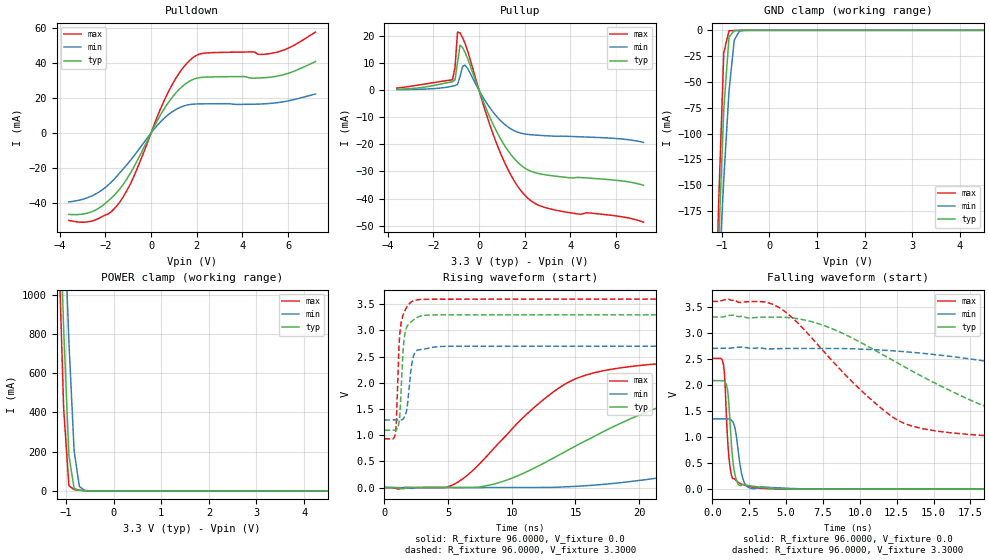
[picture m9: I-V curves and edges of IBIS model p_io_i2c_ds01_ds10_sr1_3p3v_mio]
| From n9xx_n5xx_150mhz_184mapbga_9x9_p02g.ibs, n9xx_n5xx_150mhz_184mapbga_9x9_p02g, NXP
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[Model] p_io_i2c_ds01_ds10_sr1_3p3v_mio
|   Model p_io_i2c_ds01_ds10_sr1_3p3v_mio
| This model was characterised for following simulation conditions:
| External (pad) voltage:
|   - Typ: 3.3V,   - Min: 2.7V,   - Max: 3.6V
| Library cells for typ/min/max conditions are connected as defined below:
|  pad - External Pad
|  ipp_do_lv - Core Input
|  ipp_obe_lv - Output Buffer Enable
|  IOGC - NC
|  REFH3V3 - REFH3V3
|  REFL3V3 - REFL3V3
|  ZI - NC
|  abut_ncal_vddio[1] - vddio
|  abut_ncal_vddio[2] - vddio
|  abut_ncal_vddio[3] - vssio
|  abut_ncal_vddio[4] - vddio
|  abut_ncal_vddio[5] - vddio
|  abut_ncal_vddio[6] - vssio
|  abut_pcal_vddio[1] - vssio
|  abut_pcal_vddio[2] - vssio
|  abut_pcal_vddio[3] - vddio
|  abut_pcal_vddio[4] - vssio
|  abut_pcal_vddio[5] - vssio
|  abut_pcal_vddio[6] - vddio
|  ipp_do_1p8v - ipp_do_1p8v
|  ipp_dse_lv[0] - vdd_lv
|  ipp_dse_lv[1] - 0
|  ipp_eftd_lv - NC
|  ipp_ina_mux_vddio - NC
|  ipp_ina_mux_vddio[0] - NC
|  ipp_ina_mux_vddio[1] - NC
|  ipp_ina_r0_vddio - NC
|  ipp_ina_r0a_vddio - NC
|  ipp_ina_r0b_vddio - NC
|  ipp_ina_r0c_vddio - NC
|  ipp_ina_r0d_vddio - NC
|  ipp_ina_r0e_vddio - NC
|  ipp_ina_r0f_vddio - NC
|  ipp_ina_r300_vddio - NC
|  ipp_ina_r300a_vddio - NC
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Model_type I/O
Polarity   Non-Inverting
Enable   Active-High
Vinl =   0.9900V
Vinh =   2.3100V
Vmeas =  1.6500V
Cref =   30.0000pF
Rref =   1.0000M
Vref =   3.3000V
C_comp   1.4149pF   1.3702pF   1.4746pF
|C_comp_pullup   0.5856pF   0.6310pF   0.5570pF
|C_comp_pulldown   0.7313pF   0.7412pF   0.7168pF
[Model Spec]
| variable   typ   min   max
Vinh   2.3100V   1.8900V   2.5200V
Vinl   0.9900V   0.8100V   1.0800V
[Temperature Range]   25.0000   0.1250k   -40.0000
[Voltage Range]   3.3000V   2.7000V   3.6000V
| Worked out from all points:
|   slope of the pulldown table from 0 to 0.495 V, typ, clamps not added: 40.9 ohm
|   slope of the pullup table from 0 to 0.495 V, typ, clamps not added: 47.8 ohm
|   GND clamp passes 1 mA (typ) near -0.75 V on its own axis
|   POWER clamp passes 1 mA (typ) near -0.57 V on its own axis
|   rising waveform, R_fixture 96.0000, V_fixture 0.0: 20-80 % time 11.3ns typ, 24.1ns min, 6.75ns max; typ from 0 V to 2.08 V
|   rising waveform, R_fixture 96.0000, V_fixture 3.3000: 20-80 % time 312ps typ, 386ps min, 297ps max; typ from 1.09 V to 3.3 V
|   falling waveform, R_fixture 96.0000, V_fixture 0.0: 20-80 % time 335ps typ, 413ps min, 303ps max; typ from 2.08 V to 0 V
|   falling waveform, R_fixture 96.0000, V_fixture 3.3000: 20-80 % time 9.27ns typ, 20.2ns min, 5.63ns max; typ from 3.3 V to 1.09 V
[Pulldown]
|Voltage   I(typ)   I(min)   I(max)
-3.6V     -46.61mA   -39.46mA   -50.05mA
-2.5V     -44.55mA   -35.45mA   -50.06mA
-1.84V    -38.47mA   -29.36mA   -46.05mA
-1.4V     -32.52mA   -23.26mA   -40.08mA
-850mV    -21.84mA   -14.86mA   -27.68mA
140mV     3.705mA    2.322mA    4.92mA
800mV     18.17mA    10.88mA    24.6mA
1.35V     26.36mA    15.01mA    36.38mA
1.79V     30.32mA    16.37mA    42.59mA
2.45V     31.91mA    16.62mA    45.72mA
5.42V     32.23mA    17.11mA    45.87mA
7.2V      40.82mA    22.25mA    57.64mA
[Pullup]
|Voltage   I(typ)   I(min)   I(max)
-3.6V     399uA      213.2uA    834.8uA
-1.16V    3.164mA    1.529mA    3.876mA
-1.05V    3.864mA    1.713mA    8.441mA
-940mV    10.38mA    2.174mA    21.51mA
-830mV    16.66mA    5.095mA    21.21mA
-720mV    15.81mA    8.818mA    19.46mA
-610mV    13.99mA    9.291mA    17.29mA
820mV     -16.01mA   -10.12mA   -20.75mA
1.48V     -24.65mA   -14.67mA   -32.61mA
2.03V     -28.87mA   -16.18mA   -39mA
3.24V     -31.63mA   -16.93mA   -44.08mA
7.2V      -35.1mA    -19.26mA   -48.74mA
[GND_clamp]
|Voltage   I(typ)   I(min)   I(max)
-3.6V     -4.327A    -3.181A    -5.901A
-1.18V    -358.9mA   -350.6mA   -379.3mA
-1.07V    -208.2mA   -244.2mA   -170.8mA
-960mV    -76.59mA   -144.3mA   -21.58mA
-850mV    -6.561mA   -58.74mA   -511.4uA
-740mV    -273.3uA   -9.382mA   -185.3uA
-630mV    -73.8uA    -593.1uA   -77.52uA
-410mV    -3.432uA   -9.016uA   -2.104uA
7.2V      0A         0A         0A
[POWER_clamp]
|Voltage   I(typ)   I(min)   I(max)
-3.6V     20.44A     18.76A     22.48A
-1.16V    1.647A     2.216A     1.289A
-1.05V    823.6mA    1.482A     419.2mA
-940mV    180.4mA    758.9mA    26.72mA
-830mV    12.56mA    202.9mA    6.794mA
-720mV    3.422mA    22.23mA    3.58mA
-610mV    1.373mA    2.923mA    1.344mA
7.2V      0A         0A         0A
[Ramp]
| variable   typ   min   max
dV/dt_r  1.2490/11.3046n   0.8051/24.1205n   1.5058/6.7522n
dV/dt_f  1.3240/9.2748n   0.8436/20.1848n   1.6013/5.6265n
R_load = 96.0000
[Rising Waveform]
R_fixture= 96.0000
V_fixture= 0.0
V_fixture_min= 0.0
V_fixture_max= 0.0
|time   V(typ)   V(min)   V(max)
0s        2.177nV    161nV      7.426nV
5ns       -101.8uV   -267.9uV   13.18mV
6.655ns   928.3uV    -41.54uV   264.6mV
8.959ns   90.23mV    -31.91uV   845.4mV
14.59ns   739.2mV    16.63mV    2.03V
21.47ns   1.525V     181.3mV    2.363V
31.2ns    1.902V     558.5mV    2.462V
42.19ns   2.009V     950.9mV    2.494V
53.4ns    2.05V      1.145V     2.504V
134.5ns   2.082V     1.342V     2.51V
[Rising Waveform]
R_fixture= 96.0000
V_fixture= 3.3000
V_fixture_min= 2.7000
V_fixture_max= 3.6000
|time   V(typ)   V(min)   V(max)
0s        1.093V     1.29V      931.2mV
869.1ps   1.093V     1.29V      1.056V
941.5ps   1.102V     1.29V      1.305V
1.188ns   1.325V     1.29V      2.877V
1.389ns   2.313V     1.296V     3.235V
1.525ns   2.79V      1.325V     3.334V
1.717ns   3.047V     1.445V     3.433V
2.22ns    3.19V      2.454V     3.56V
2.775ns   3.271V     2.633V     3.591V
134.5ns   3.3V       2.7V       3.6V
[Falling Waveform]
R_fixture= 96.0000
V_fixture= 0.0
V_fixture_min= 0.0
V_fixture_max= 0.0
|time   V(typ)   V(min)   V(max)
0s        2.082V     1.348V     2.51V
752.7ps   2.081V     1.348V     2.387V
841.1ps   2.065V     1.348V     2.118V
1.047ns   1.864V     1.349V     889.7mV
1.333ns   707.7mV    1.312V     233.9mV
1.664ns   148.6mV    941.7mV    149.5mV
1.921ns   67.98mV    392.5mV    104.5mV
2.178ns   86.63mV    119.9mV    77.71mV
3.439ns   29.38mV    42.48mV    13.78mV
134.5ns   155.1nV    3.236uV    24.62nV
[Falling Waveform]
R_fixture= 96.0000
V_fixture= 3.3000
V_fixture_min= 2.7000
V_fixture_max= 3.6000
|time   V(typ)   V(min)   V(max)
0s        3.3V       2.7V       3.6V
4.025ns   3.3V       2.69V      3.552V
7.076ns   3.185V     2.7V       2.793V
12.56ns   2.419V     2.647V     1.324V
18.04ns   1.643V     2.475V     1.036V
21.01ns   1.397V     2.346V     994.9mV
25.71ns   1.258V     2.121V     963.2mV
35.83ns   1.155V     1.674V     940.5mV
46.32ns   1.12V      1.474V     934.3mV
134.5ns   1.093V     1.294V     931.2mV
